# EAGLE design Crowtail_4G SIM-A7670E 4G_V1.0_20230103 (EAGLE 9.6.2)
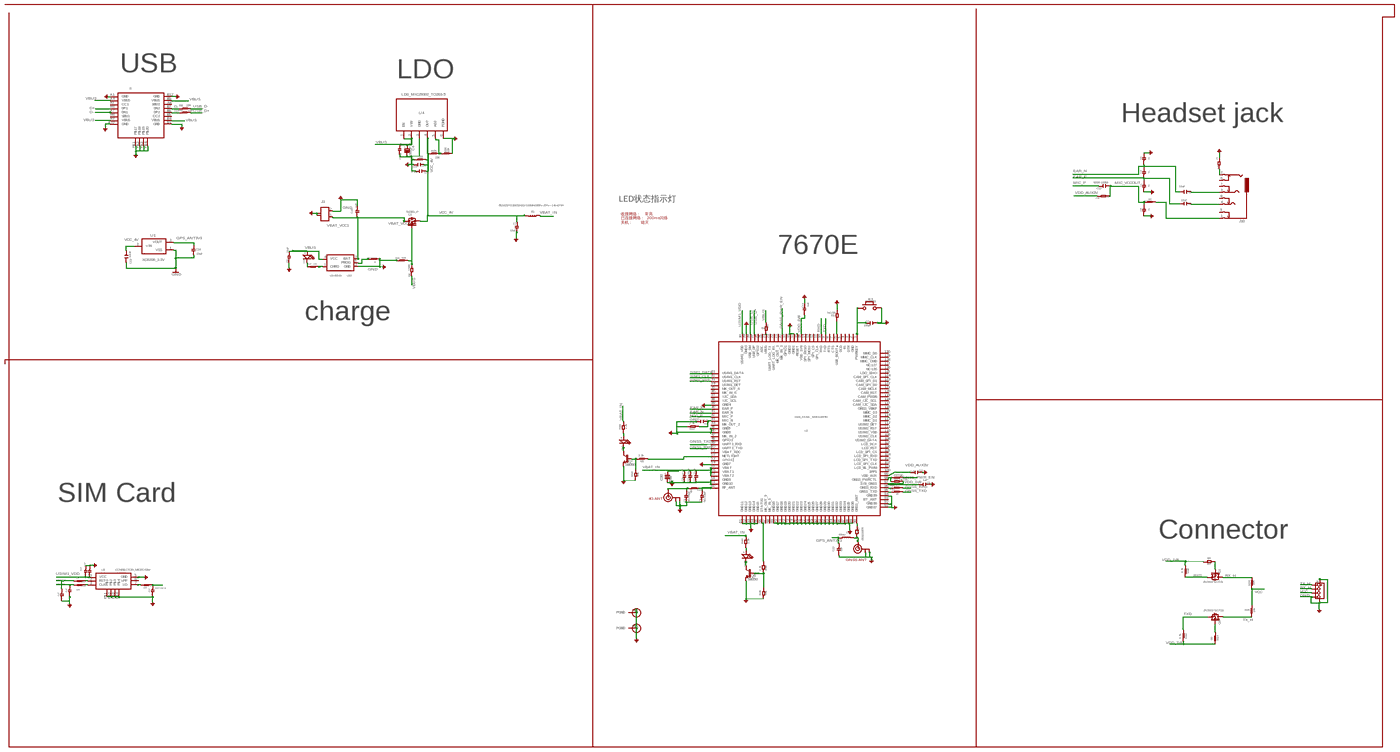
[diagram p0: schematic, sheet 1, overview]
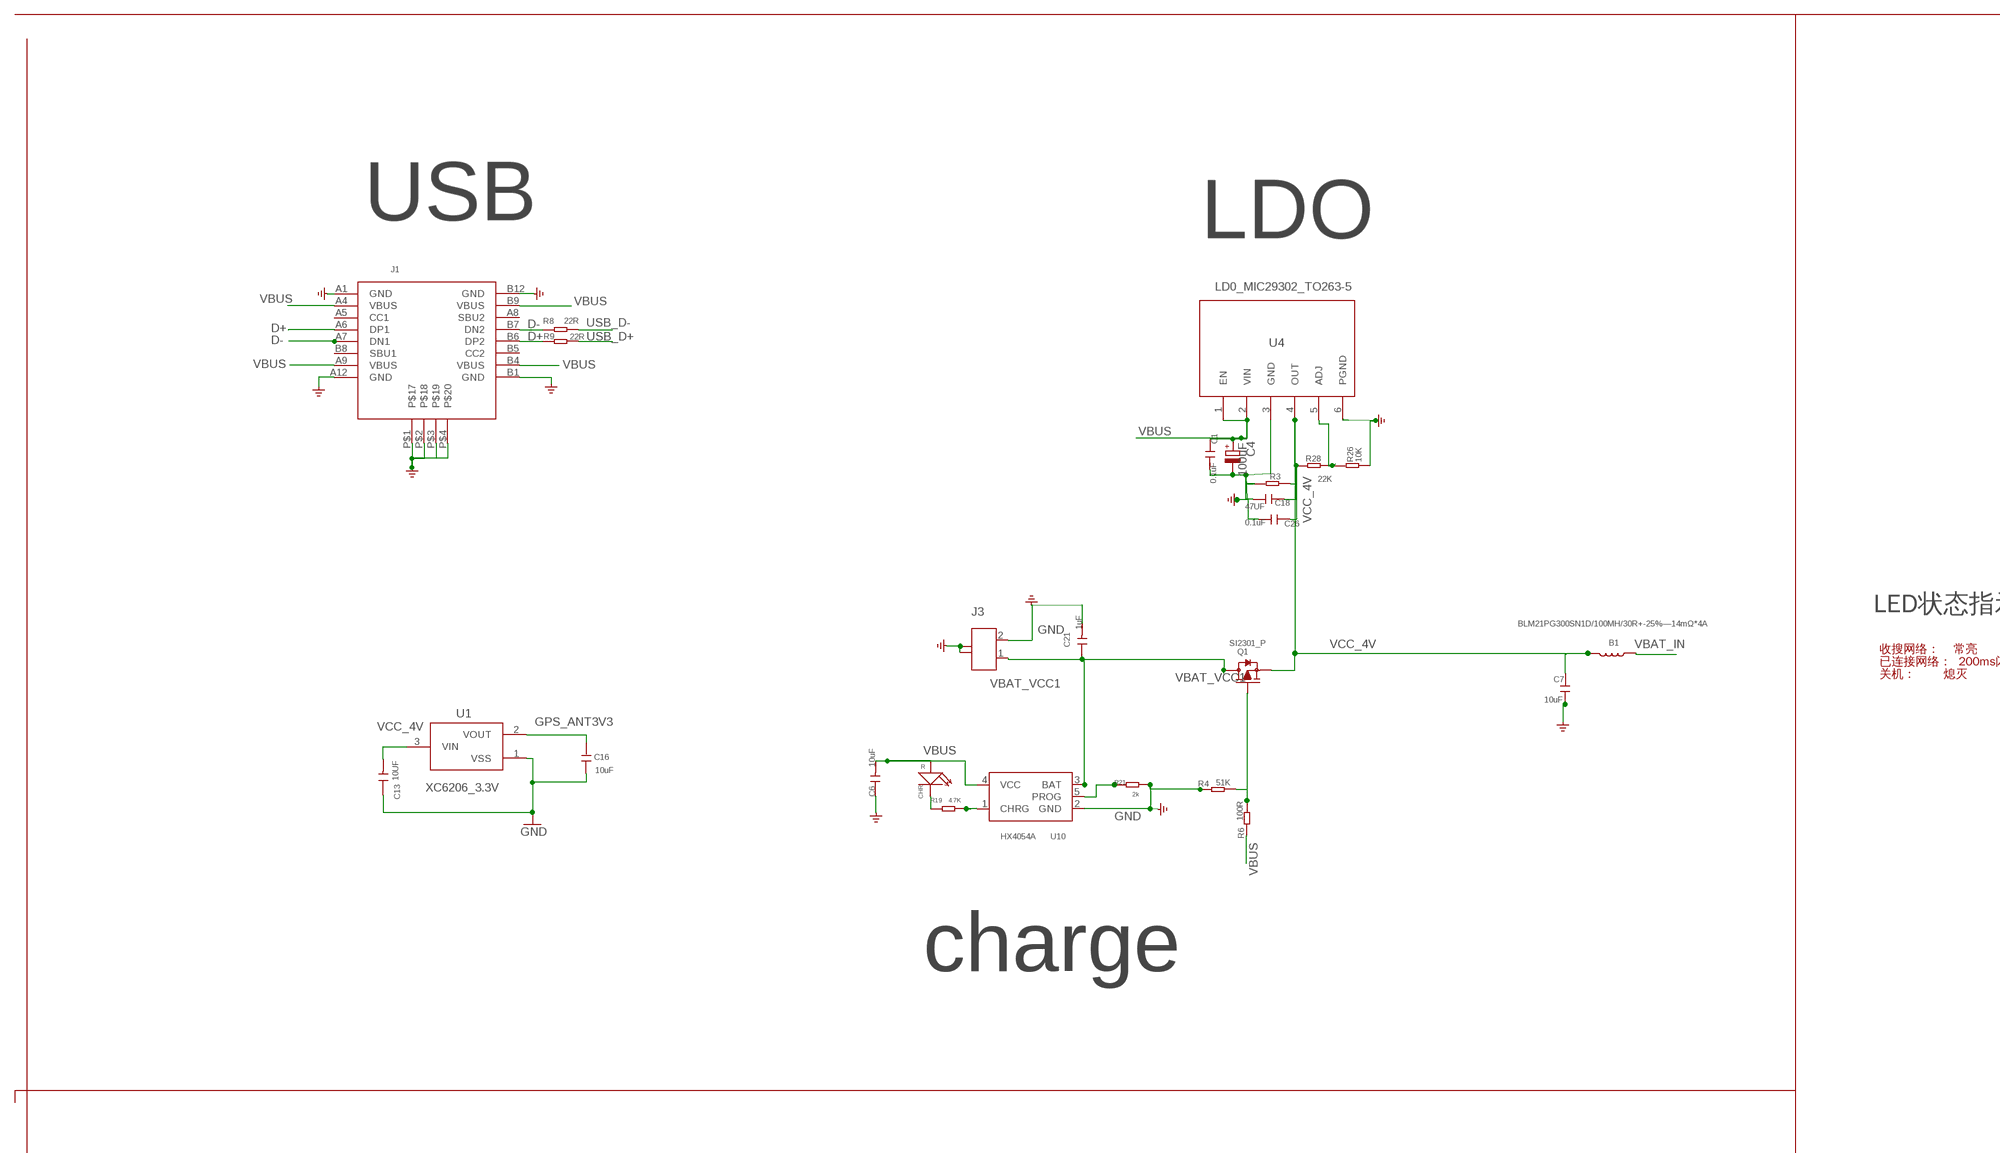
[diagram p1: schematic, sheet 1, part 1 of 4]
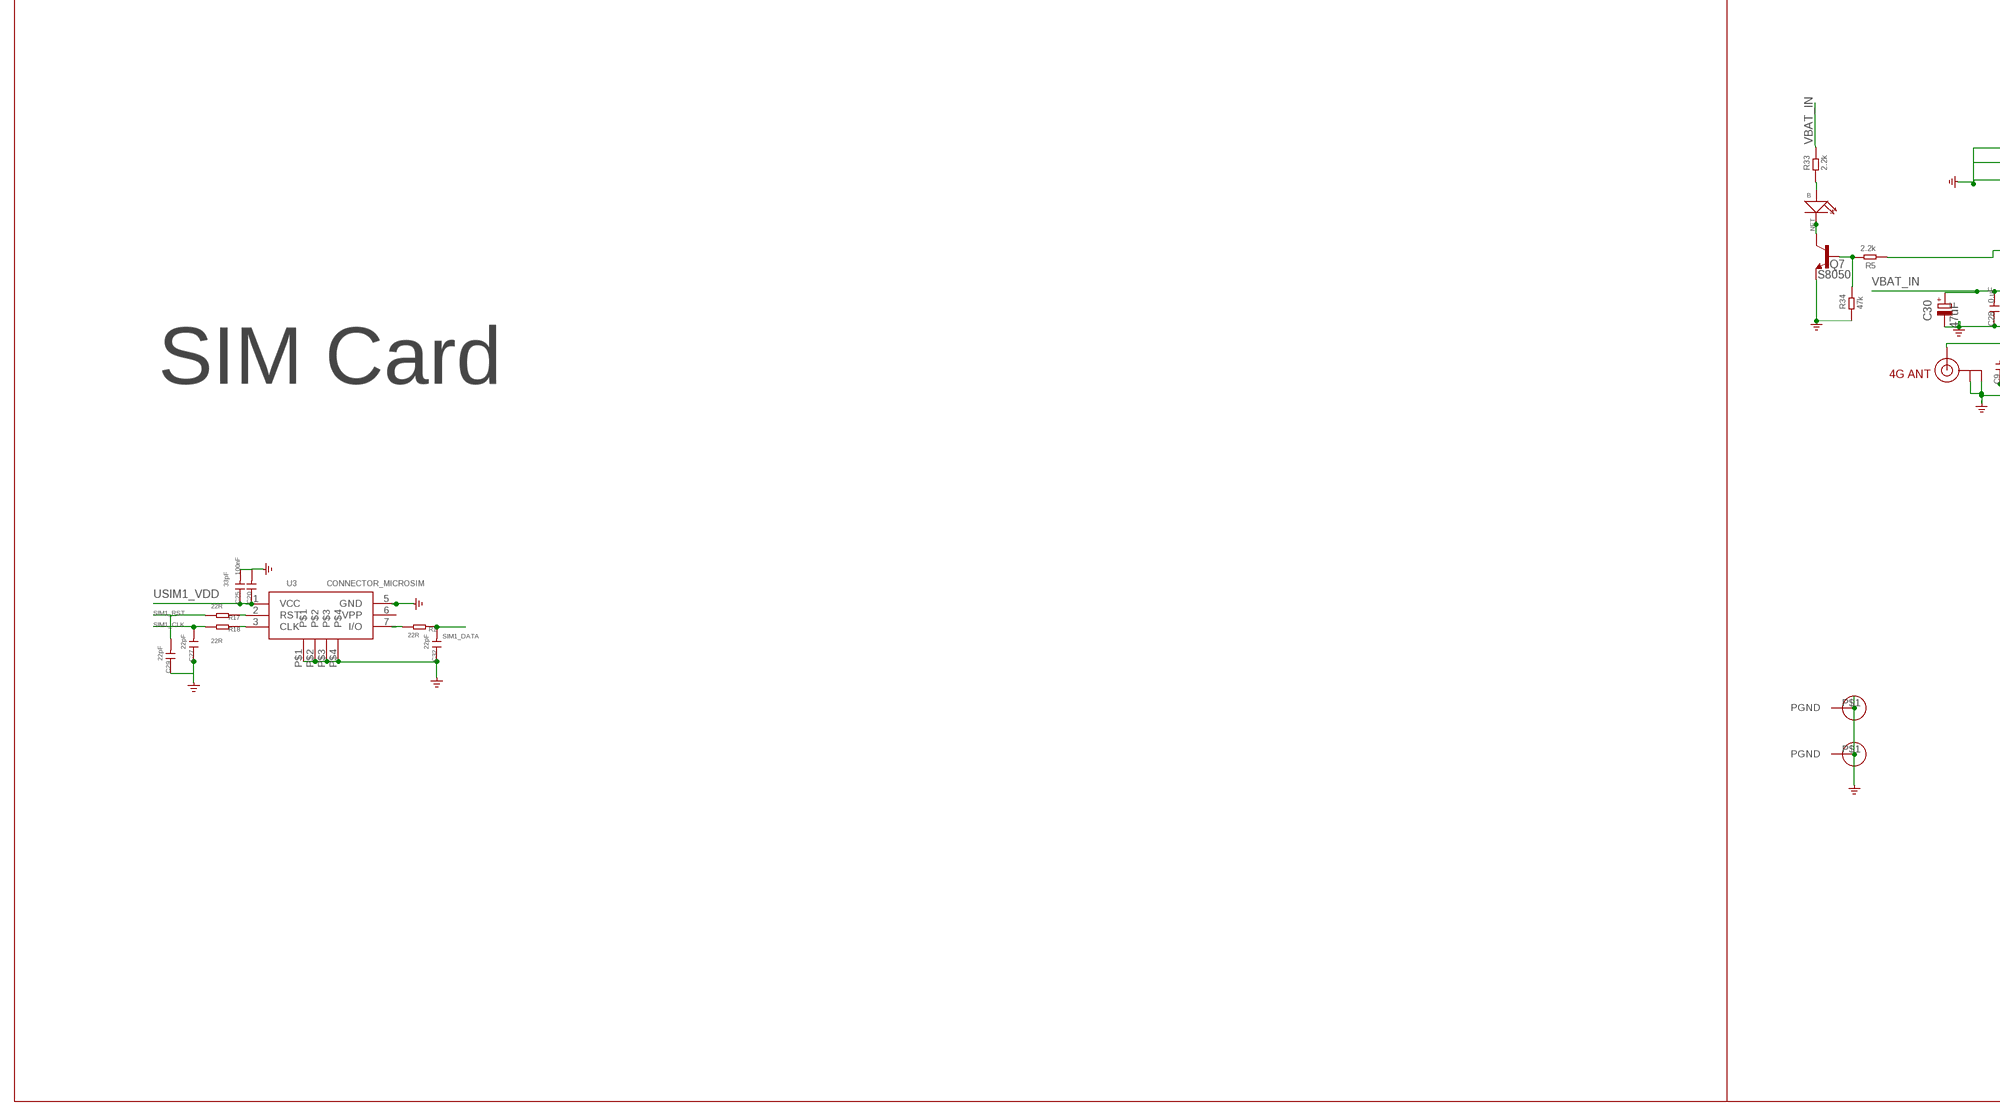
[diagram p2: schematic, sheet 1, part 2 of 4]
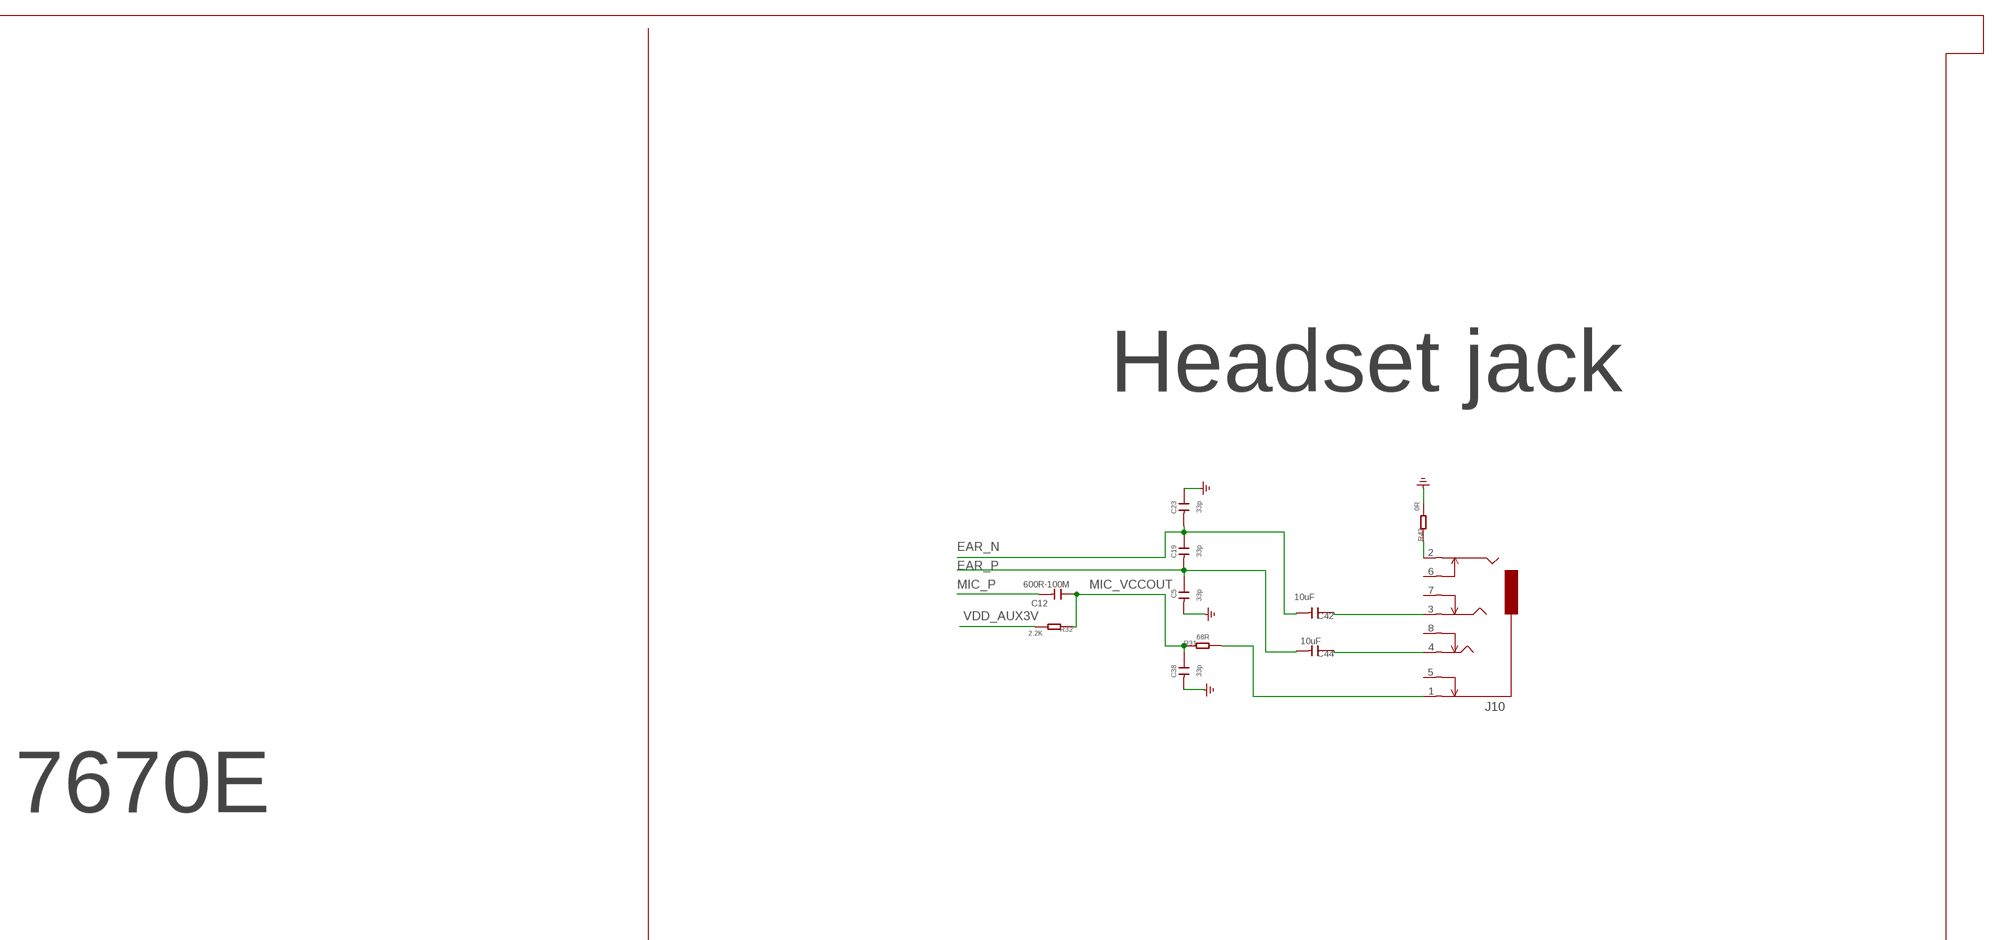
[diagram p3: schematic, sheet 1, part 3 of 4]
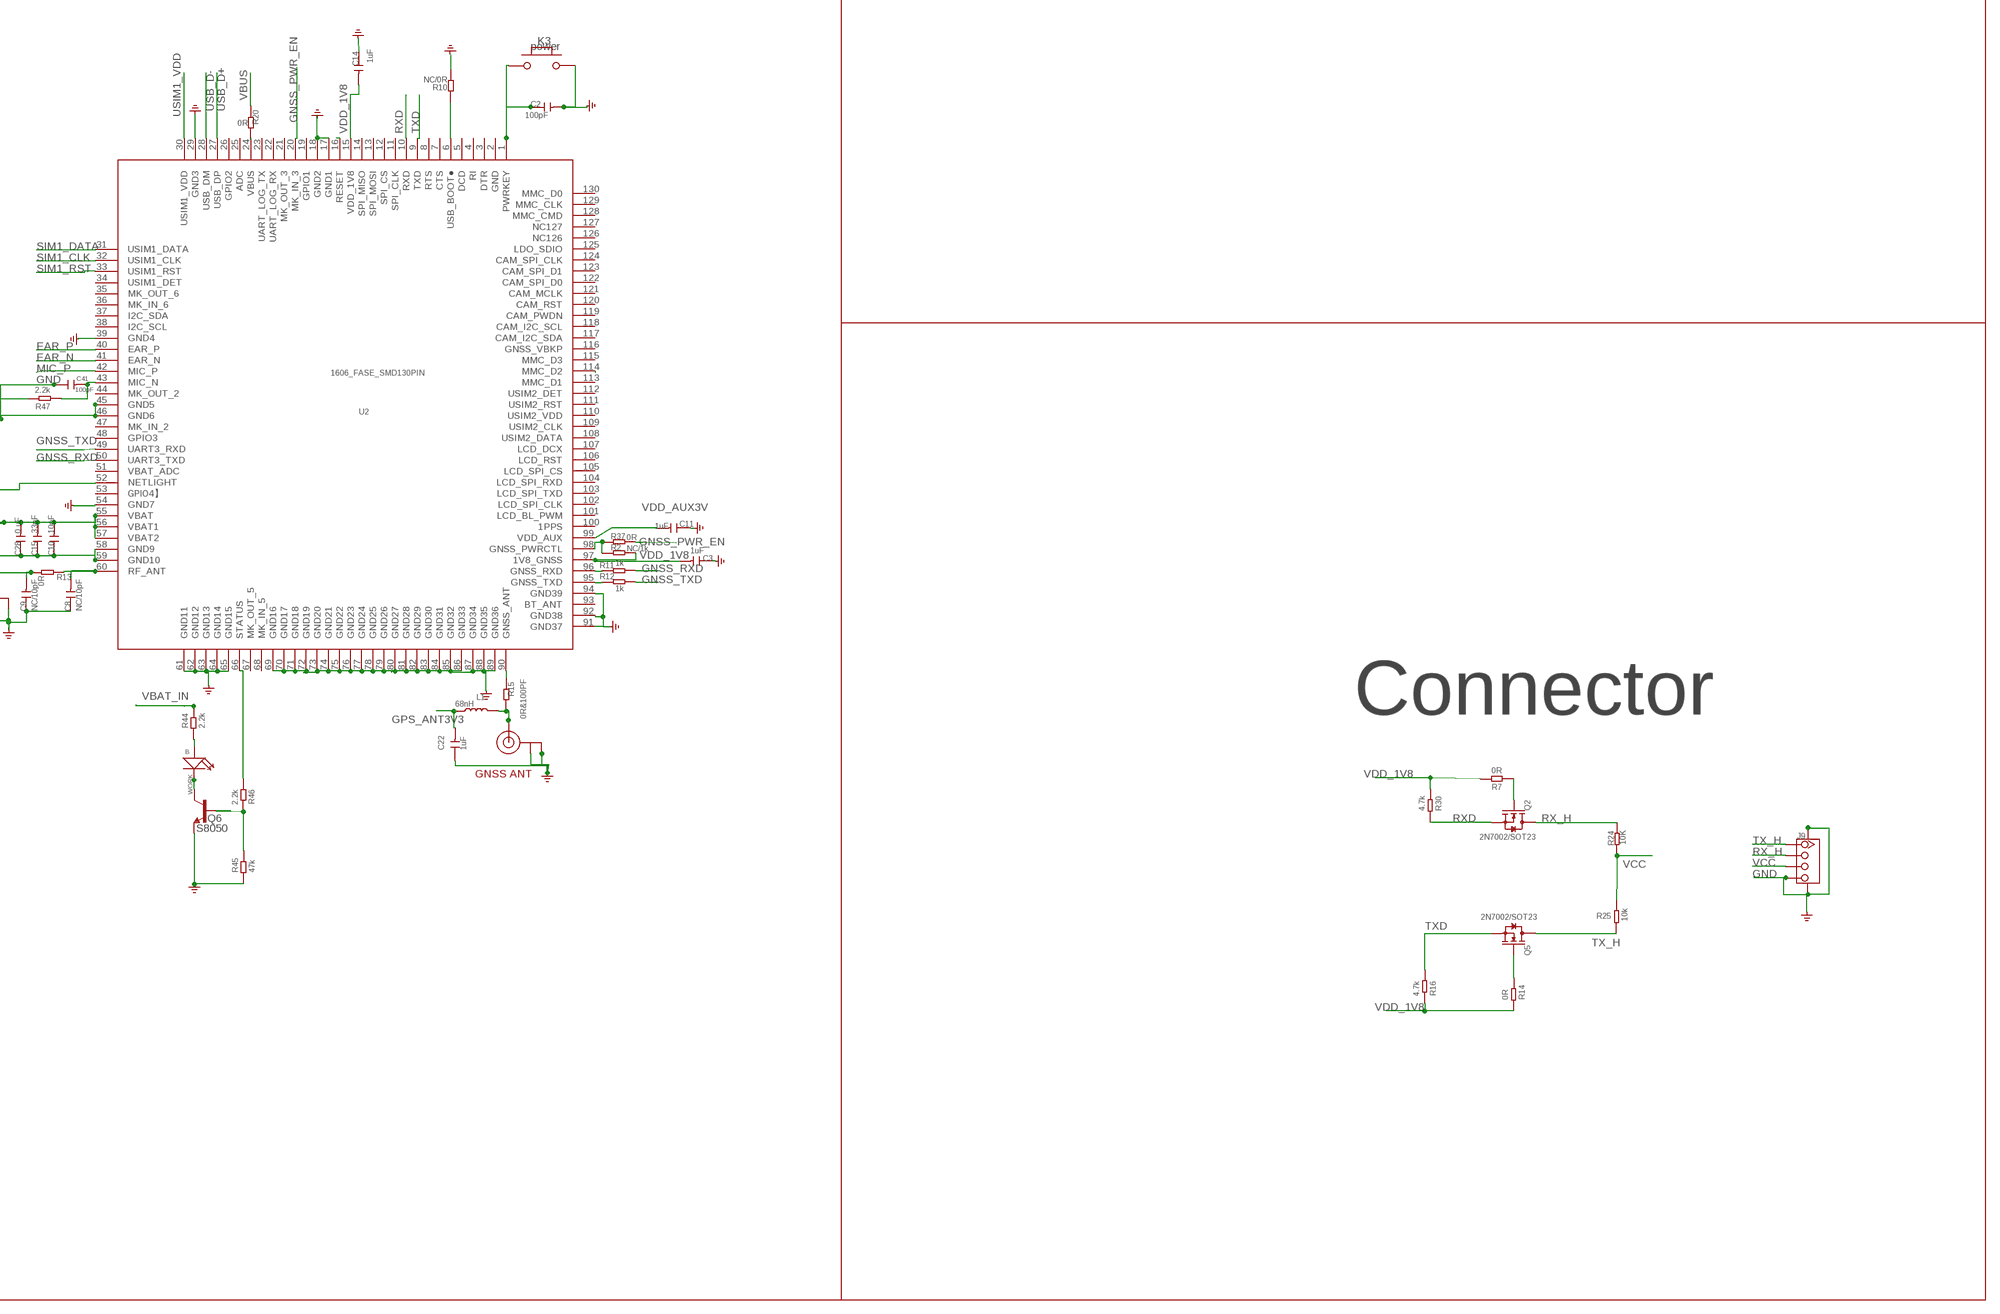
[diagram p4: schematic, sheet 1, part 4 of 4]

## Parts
B1  BLM21PG300SN1D/100MH/30R+-25%—14mΩ*4A  L0805  [0805@1]
C1  0.1uF  C0603  [0603]
C2  100pF  C-0603  [C0603]
C3  1uF  C-0603  [C0603]
C4  100uF  CPOL-EUSMCB  [SMC_B]
C5  33p  C-0603  [C0603]
C6  10uF  C-0603  [C0603]
C7  10uF  C0603  [0603]
C8  NC/10pF  C-0603  [C0603]
C9  NC/10pF  C-0603  [C0603]
C10  10pF  C-0603  [C0603]
C11  1uF  C-0603  [C0603]
C12  600R-100M  C-0603  [C0603]
C13  10UF  C-0603  [C0603]
C14  1uF  C-0603  [C0603]
C15  33pF  C-0603  [C0603]
C16  10uF  C0603  [0603]
C18  47UF  C0805  [0805]
C19  33p  C-0603  [C0603]
C20  100nF  C-0603  [C0603]
C21  1uF  C-0603  [C0603]
C22  1uF  C-0603  [C0603]
C23  33p  C-0603  [C0603]
C25  33pF  C-0603  [C0603]
C26  0.1uF  C0603  [0603]
C27  22pF  C-0603  [C0603]
C28  0.uF  C-0603  [C0603]
C29  22pF  C-0603  [C0603]
C30  47uF  CPOL-EUSMCB  [SMC_B]
C32  22pF  C-0603  [C0603]
C38  33p  C-0603  [C0603]
C41  100pF  C-0603  [C0603]
C42  10uF  C-0603  [C0603]
C44  10uF  C-0603  [C0603]
CHR  R  007-LED0603  [D0603]
J1  TYPEC-3.0-16P-SMD  [TYPEC-3.0-16P-SMD]
J3  PH2.0_2P  [PH2.0_2P]
J4  IPEX一代  U.FL  [U.FL]
J6  IPEX一代  U.FL  [U.FL]
J9  TWIG-4P-2.0-SMD-FEMALE-REINFORCE'DD'  [4P-SMD-2.0]
J10  AUDIO-8P'PJ-3536-L6S'  [8P-3.5-SMD]
K3  BUTTON  PB157  [157SW]
L1  68nH  BL_0603  [BL_0603]
NET  B  007-LED0603  [D0603]
Q1  SI2301_P  DISCRETE_MOSFET-PSOT23  [DISCRETE_SOT23]
Q2  2N7002/SOT23  MOSFET-N'SOT23'  [SOT23]
Q5  2N7002/SOT23  MOSFET-N'SOT23'  [SOT23]
Q6  S8050  SPARKFUN_TRANSISTOR_NPNSOT23  [SPARKFUN_SOT23]
Q7  S8050  SPARKFUN_TRANSISTOR_NPNSOT23  [SPARKFUN_SOT23]
R1  22R  R-0603  [R0603]
R2  NC/1k  DISCRETE_R-0603  [DISCRETE_R0603]
R3  NC/470R  DISCRETE_R-0603  [DISCRETE_R0603]
R4  51K  R0603  [R0603]
R5  2.2k  DISCRETE_R-0603  [DISCRETE_R0603]
R6  100R  R0603  [R0603]
R7  0R  R-0603  [R0603]
R8  22R  DISCRETE_R-0603  [DISCRETE_R0603]
R9  22R  DISCRETE_R-0603  [DISCRETE_R0603]
R10  NC/0R  DISCRETE_R-0603  [DISCRETE_R0603]
R11  1k  DISCRETE_R-0603  [DISCRETE_R0603]
R12  1k  DISCRETE_R-0603  [DISCRETE_R0603]
R13  0R  DISCRETE_R-0603  [DISCRETE_R0603]
R14  0R  R-0603  [R0603]
R15  0R&100PF  DISCRETE_R-0603  [DISCRETE_R0603]
R16  4.7k  R-0603  [R0603]
R17  22R  R-0603  [R0603]
R18  22R  R-0603  [R0603]
R19  4.7K  R-0603  [R0603]
R20  0R  DISCRETE_R-0603  [DISCRETE_R0603]
R21  2k  R-0603  [R0603]
R24  10K  R-0603  [R0603]
R25  10k  R-0603  [R0603]
R26  10K  DISCRETE_R-0603  [DISCRETE_R0603]
R28  22K  DISCRETE_R-0603  [DISCRETE_R0603]
R30  4.7k  R-0603  [R0603]
R31  68R  R-0603  [R0603]
R32  2.2K  R-0603  [R0603]
R33  2.2k  DISCRETE_R-0603  [DISCRETE_R0603]
R34  47k  DISCRETE_R-0603  [DISCRETE_R0603]
R37  0R  DISCRETE_R-0603  [DISCRETE_R0603]
R42  0R  R-0603  [R0603]
R44  2.2k  DISCRETE_R-0603  [DISCRETE_R0603]
R45  47k  DISCRETE_R-0603  [DISCRETE_R0603]
R46  2.2k  DISCRETE_R-0603  [DISCRETE_R0603]
R47  2.2k  DISCRETE_R-0603  [DISCRETE_R0603]
U1  XC6206_3.3V  XC6206  [SOT-23]
U2  1606_FASE_SMD130PIN  [1606_FASE_SMD130PIN]
U3  CONNECTOR_MICROSIM  [CONNECTOR_MICROSIM]
U4  LD0_MIC29302_TO263-5  [LD0_MIC29302_TO263-5]
U10  HX4054A  [HX4054A_SOT23_5]
U$37  PGND  [PGND]
U$38  PGND  [PGND]
WORK  B  007-LED0603  [D0603]

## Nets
D+: J1.A6(DP1) J1.B6(DP2) R9.1
D-: J1.A7(DN1) J1.B7(DN2) R8.1
EAR_N: C19.1 C23.2 C42.2 U2.41(EAR_N)
EAR_P: C5.1 C19.2 C44.2 U2.40(EAR_P)
GND: C1.1 C2.2 C3.1 C4.- C5.2 C6.1 C7.2 C8.1 C9.1 C10.1 C11.1 C13.1 C14.1 C15.1 C16.2 C18.1 C20.2 C21.2 C22.1 C23.1 C25.2 C26.1 C27.1 C28.1 C29.1 C30.- C32.1 C38.2 C41.1 J1.A1(GND) J1.A12(GND) J1.B1(GND) J1.B12(GND) J1.P$1 J1.P$2 J1.P$3 J1.P$4 J3.2 J3.3 J3.4 J4.P$1(GND) J4.P$2(GND) J6.P$1(GND) J6.P$2(GND) J9.4 J9.SS1 J9.SS2 K3.2 Q6.2(E) Q7.2(E) R3.2 R4.2 R10.2 R21.2 R26.2 R34.1 R42.2 R45.1 R47.2 U1.1(VSS) U2.17(GND1) U2.18(GND2) U2.29(GND3) U2.39(GND4) U2.45(GND5) U2.46(GND6) U2.54(GND7) U2.58(GND9) U2.59(GND10) U2.61(GND11) U2.62(GND12) U2.63(GND13) U2.64(GND14) U2.65(GND15) U2.69(GND16) U2.70(GND17) U2.71(GND18) U2.72(GND19) U2.73(GND20) U2.74(GND21) U2.75(GND22) U2.76(GND23) U2.77(GND24) U2.78(GND25) U2.79(GND26) U2.80(GND27) U2.81(GND28) U2.82(GND29) U2.83(GND30) U2.84(GND31) U2.85(GND32) U2.86(GND33) U2.87(GND34) U2.88(GND35) U2.89(GND36) U2.91(GND37) U2.92(GND38) U2.94(GND39) U3.5(GND) U3.P$1 U3.P$2 U3.P$3 U3.P$4 U4.3(GND) U4.6(PGND) U10.2(GND) U$37.P$1(PGND) U$38.P$1(PGND)
GNSS_PWR_EN: R37.2 U2.20(MK_IN_3)
GNSS_RXD: R11.2 U2.50(UART3_TXD)
GNSS_TXD: R12.2 U2.49(UART3_RXD)
GPS_ANT3V3: C16.1 C22.2 L1.1 U1.2(VOUT)
MIC_P: C12.2 U2.42(MIC_P)
MIC_VCCOUT: C12.1 C38.1 R31.1 R32.1
N$1: R18.1 U3.3(CLK)
N$2: R17.1 U3.2(RST)
N$3: Q1.1(G) R4.1 R6.1
N$4: Q2.1(G) R7.2
N$5: R5.1 U2.52(NETLIGHT)
N$6: U2.16(RESET)
N$7: CHR.- R19.1
N$8: R10.1 U2.6(USB_BOOT●)
N$9 [N9]: J4.P$3(SIGNAL) L1.2 R15.2
N$10: R12.1 U2.95(GNSS_TXD)
N$11: Q5.1(G) R14.2
N$12: R11.1 U2.96(GNSS_RXD)
N$13 [N13]: C8.2 R13.1 U2.60(RF_ANT)
N$15 [N15]: C9.2 J6.P$3(SIGNAL) R13.2
N$16 [N16]: R15.1 U2.90(GNSS_ANT)
N$17: Q7.1(B) R5.2 R34.2
N$18: C41.2 R47.1 U2.43(MIC_N)
N$20: R19.2 U10.1(CHRG)
N$21: J10.1 R31.2
N$22: R26.1 R28.1 U4.5(ADJ)
N$23: J10.2 R42.1
N$24: R1.2 U3.7(I/O)
N$25: R20.2 U2.24(VBUS)
N$26: C42.1 J10.3
N$27: C44.1 J10.4
N$29: R2.1 R37.1 U2.98(GNSS_PWRCTL)
N$31: R21.1 U10.5(PROG)
N$32: C2.1 K3.1 U2.1(PWRKEY)
N$35: NET.- Q7.3(C)
N$36: NET.+ R33.1
N$37: Q6.1(B) R45.2 R46.2
N$39: Q6.3(C) WORK.-
N$40: R44.1 WORK.+
N$41: R46.1 U2.66(STATUS)
RX_H: J9.2 Q2.3(D) R24.1
RXD: Q2.2(S) R30.1 U2.10(RXD)
SIM1_CLK: C27.2 R18.2 U2.32(USIM1_CLK)
SIM1_DATA: C32.2 R1.1 U2.31(USIM1_DATA)
SIM1_RST: C29.2 R17.2 U2.33(USIM1_RST)
TF_DAT2: U2.114(MMC_D2)
TX_H: J9.1 Q5.3(D) R25.1
TXD: Q5.2(S) R16.1 U2.9(TXD)
USB_D+: R9.2 U2.27(USB_DP)
USB_D-: R8.2 U2.28(USB_DM)
USIM1_VDD: C20.1 C25.1 U2.30(USIM1_VDD) U3.1(VCC)
VBAT_IN: B1.1 C10.2 C15.2 C28.2 C30.+ R33.2 R44.2 U2.55(VBAT) U2.56(VBAT1) U2.57(VBAT2)
VBAT_VCC1: C21.1 J3.1 Q1.3(D) U10.3(BAT)
VBUS: C1.2 C4.+ C6.2 CHR.+ J1.A4(VBUS) J1.A9(VBUS) J1.B4(VBUS) J1.B9(VBUS) R6.2 R20.1 U4.1(EN) U4.2(VIN) U10.4(VCC)
VCC: J9.3 R24.2 R25.2
VCC_4V: B1.2 C7.1 C13.2 C18.2 C26.2 Q1.2(S) R3.1 R28.2 U1.3(VIN) U4.4(OUT)
VDD_1V8: C3.2 C14.2 R2.2 R7.1 R14.1 R16.2 R30.2 U2.15(VDD_1V8) U2.97(1V8_GNSS)
VDD_AUX3V: C11.2 R32.2 U2.99(VDD_AUX)
Unconnected: J1.A5(CC1) J1.A8(SBU2) J1.B5(CC2) J1.B8(SBU1) J10.5 J10.6 J10.7 J10.8 U2.2(GND) U2.3(DTR) U2.4(RI) U2.5(DCD) U2.7(CTS) U2.8(RTS) U2.11(SPI_CLK) U2.12(SPI_CS) U2.13(SPI_MOSI) U2.14(SPI_MISO) U2.19(GPIO1) U2.21(MK_OUT_3) U2.22(UART_LOG_RX) U2.23(UART_LOG_TX) U2.25(ADC) U2.26(GPIO2) U2.34(USIM1_DET) U2.35(MK_OUT_6) U2.36(MK_IN_6) U2.37(I2C_SDA) U2.38(I2C_SCL) U2.44(MK_OUT_2) U2.47(MK_IN_2) U2.48(GPIO3) U2.51(VBAT_ADC) U2.53(GPIO4】) U2.67(MK_OUT_5) U2.68(MK_IN_5) U2.93(BT_ANT) U2.100(1PPS) U2.101(LCD_BL_PWM) U2.102(LCD_SPI_CLK) U2.103(LCD_SPI_TXD) U2.104(LCD_SPI_RXD) U2.105(LCD_SPI_CS) U2.106(LCD_RST) U2.107(LCD_DCX) U2.108(USIM2_DATA) U2.109(USIM2_CLK) U2.110(USIM2_VDD) U2.111(USIM2_RST) U2.112(USIM2_DET) U2.113(MMC_D1) U2.115(MMC_D3) U2.116(GNSS_VBKP) U2.117(CAM_I2C_SDA) U2.118(CAM_I2C_SCL) U2.119(CAM_PWDN) U2.120(CAM_RST) U2.121(CAM_MCLK) U2.122(CAM_SPI_D0) U2.123(CAM_SPI_D1) U2.124(CAM_SPI_CLK) U2.125(LDO_SDIO) U2.126(NC126) U2.127(NC127) U2.128(MMC_CMD) U2.129(MMC_CLK) U2.130(MMC_D0) U3.6(VPP)

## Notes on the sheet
- USB | LDO
- Headset jack
- LED状态指示灯
- 收搜网络：    常亮 
  已连接网络：  200ms闪烁
  关机：        熄灭
- 7670E
- power
- charge
- 4G ANT
- SIM Card
- Connector
- GNSS ANT

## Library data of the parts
B1 = Discrete:L*
C1 C7 C16 C26 = cooper:C0603
C2 C3 C5 C6 C8-C15 C19-C23 C25 C27-C29 C32 C38 C41 C42 C44 = Discrete:C*: Ceramic Capacitors
C4 C30 = rcl:CPOL-EU: POLARIZED CAPACITOR, European symbol
C18 = cooper:C0805
CHR NET WORK = Discrete:007-LED*
J1 = A_xbj:TYPEC-3.0-16P-SMD
J3 = A_xbj:PH2.0_2P
J4 J6 = SparkFun2:U.FL
J9 = Connector:TWIG-4P-2.0-SMD-FEMALE-REINFORCE
J10 = template:AUDIO-8P
K3 = MySMD:PB157
L1 = untitled:BL_0603
Q1 = untitled:DISCRETE_MOSFET-P: IRLL014: http://www.vishay.com/docs/91319/sihll014.pdf
Q2 Q5 = Discrete:MOSFET-N: IRLL014: http://www.vishay.com/docs/91319/sihll014.pdf
Q6 Q7 = Adafruit_HUZZAH32_ESP32_Feather:SPARKFUN_TRANSISTOR_NPN: Transistor NPN BJT configuration in SOT23 package. MMBT2222 is the common NPN we use. Double check BCE configuration again layout.
R1 R7 R14 R16-R19 R21 R24 R25 R30-R32 R42 = Discrete:R*
R2 R5 R8 R9 R11 R12 R33 R34 R37 R44-R47 = Crowtail-_LED-V2.0-20190615-01:DISCRETE_R*
R3 R10 R13 R15 R20 R26 R28 = A9G:DISCRETE_R*
R4 R6 = cooper:R0603
U1 = self:XC6206
U2 = A7670E_FASE_SMD124PIN:1606_FASE_SMD130PIN
U3 = MINISIM_MUPC713-23_6PIN:CONNECTOR_MICROSIM
U4 = LD0_MIC29302_TO263-5:LD0_MIC29302_TO263-5
U10 = ESP32-S3-WROOM-2-N32R8V1:HX4054A
U$37 U$38 = QC:PGND

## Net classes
0 default: width 0.152 mm, drill 0.3 mm, clearance 0.152 mm
1 N9: drill 0.533 mm, clearance 0.533 mm to class 0, clearance 0.533 mm
2 N13: drill 0.533 mm, clearance 0.533 mm to class 0, clearance 0.533 mm
3 N15: drill 0.533 mm, clearance 0.533 mm to class 0, clearance 0.533 mm
4 N16: clearance 0.254 mm to class 0, clearance 0.254 mm

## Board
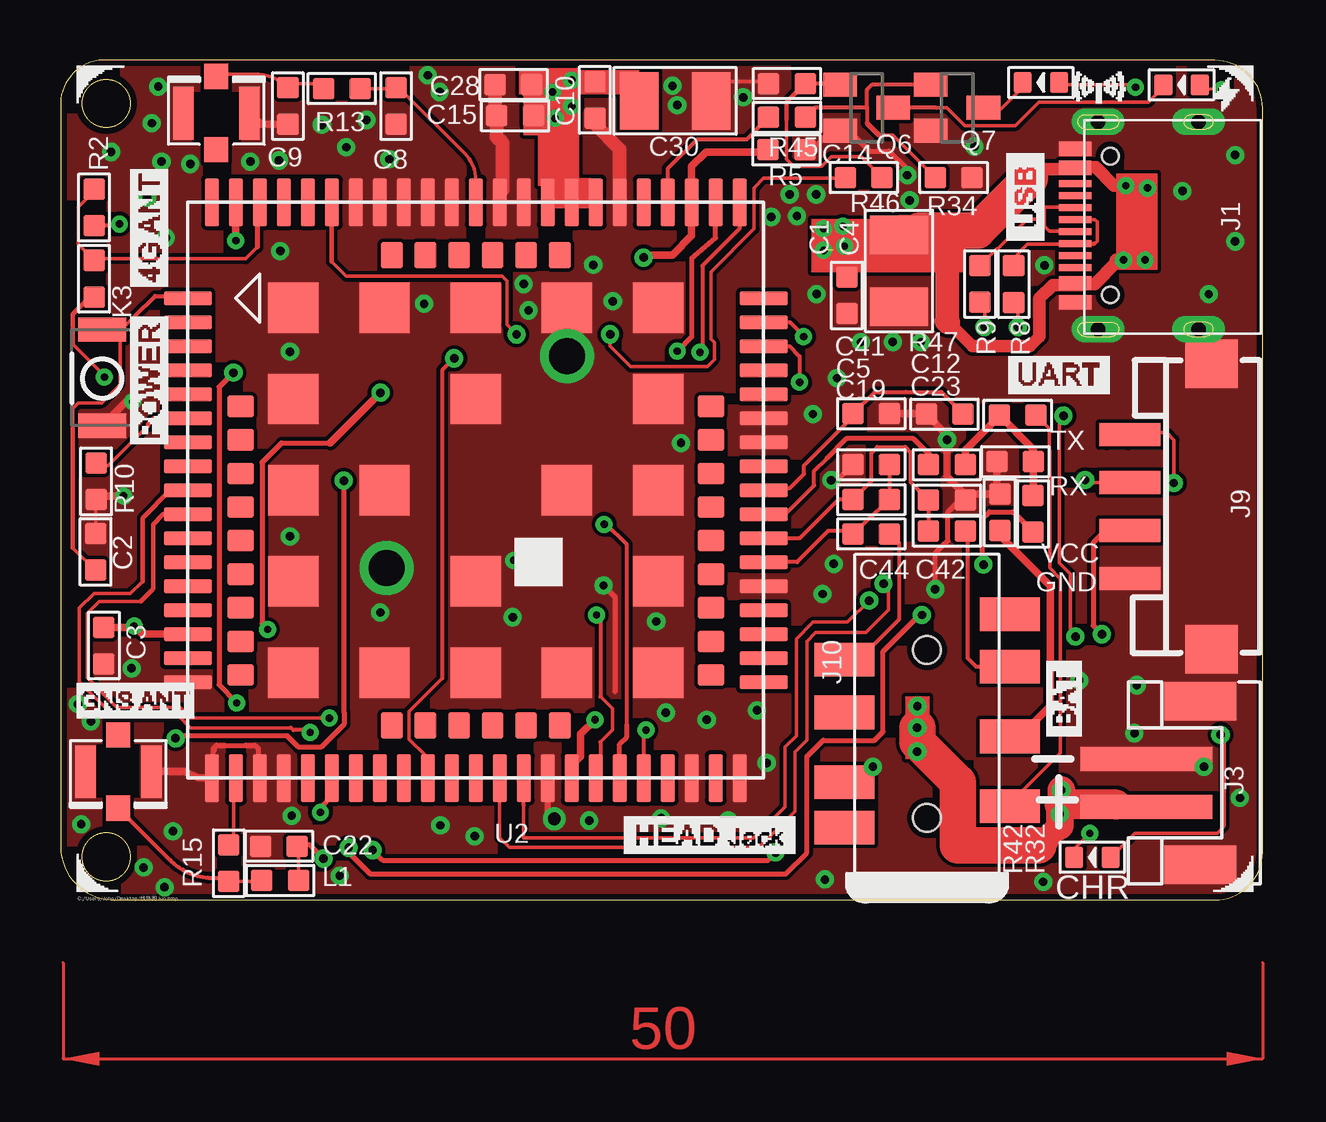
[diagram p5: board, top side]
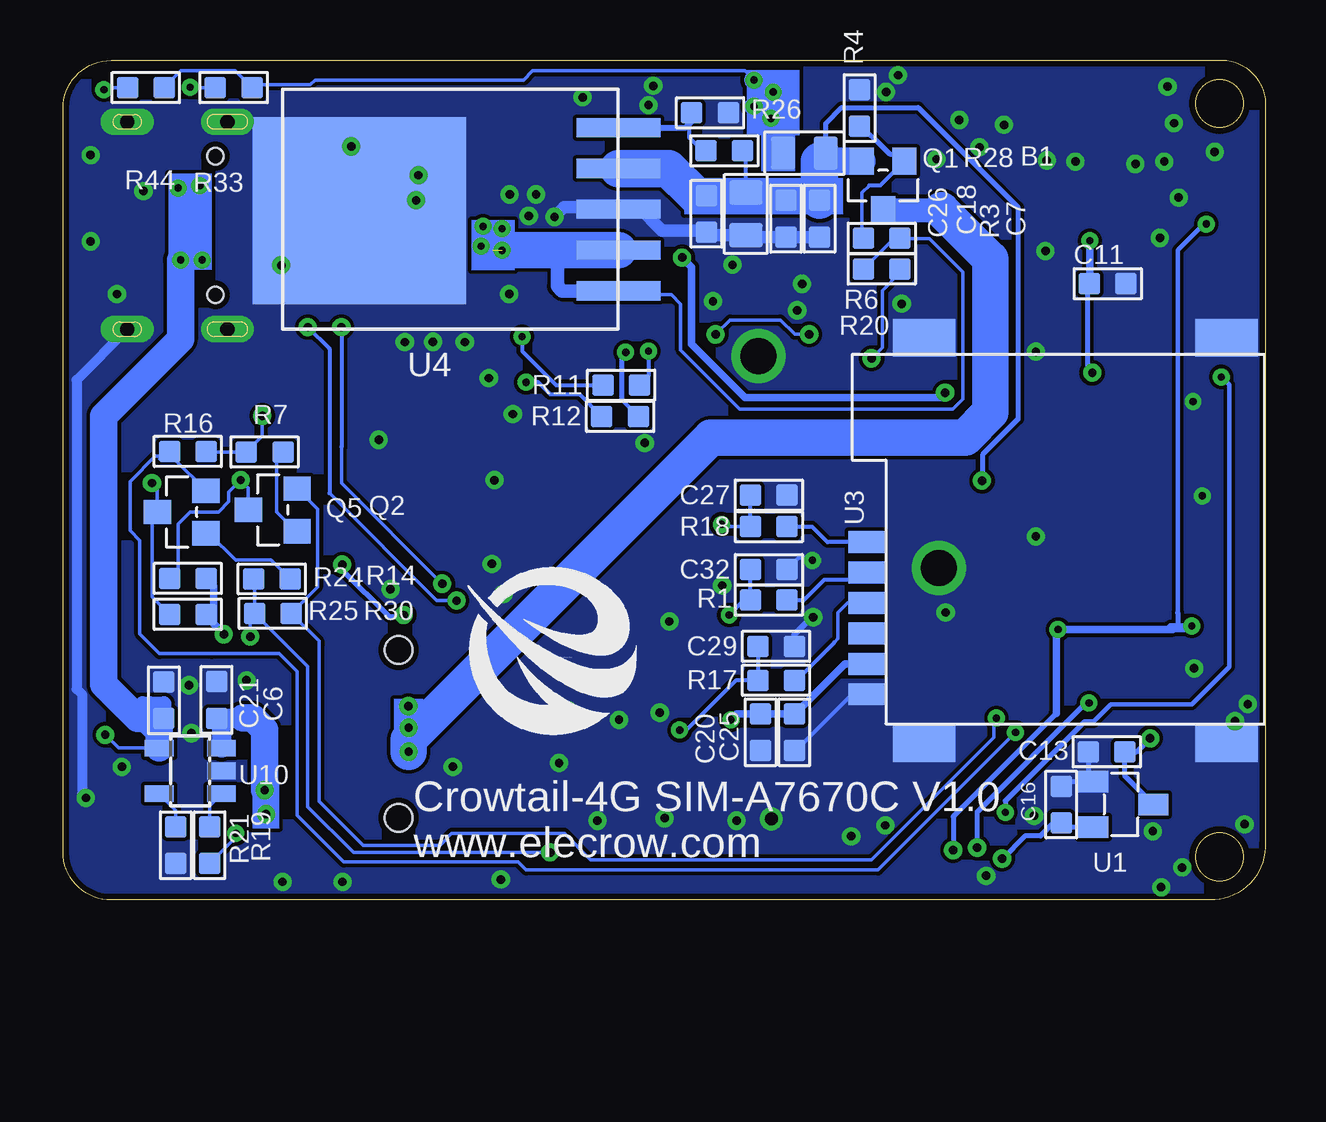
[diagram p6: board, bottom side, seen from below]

Size 50.1 x 35.02 mm. Coordinates in mm from the lower left corner, seen from the top.
Outline: 0,33.4 0,2.4 arc90 2.1,0 48.1,0 arc90 50.1,2 50.1,33 arc90 48.1,35 2.1,35 arc90 0,33.4
Outline: circle at 1.9,33.2 radius 1
Outline: circle at 1.9,1.8 radius 1
Copper layers (1*16): Top 0.035mm / dielectric 1.5mm / Bottom 0.035mm
Design rules "default *": minimum track width 6mil, minimum drill 0.3mm, track to track 6mil, track to pad 6mil, pad to pad 6mil, via to via 6mil, smd to smd 6mil, copper to edge 10mil, drill to drill 6mil, minimum pad ring 10mil, minimum via ring 8mil, stop-mask expansion 4mil, vias tented up to drill 40mil, thermal gap 10mil
tRestrict: area 5.5,31.5 to 7.5,33.7; area 1.5,4.3 to 3.3,6.5

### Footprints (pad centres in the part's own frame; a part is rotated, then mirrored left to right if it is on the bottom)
0805@1 = smd 1.016 x 1.397: 1 -0.889,0; 2 0.889,0
0603 = smd 0.889 x 0.889: 1 -0.762,0; 2 0.762,0
C0603 = smd 0.889 x 0.889: 1 -0.762,0; 2 0.762,0
SMC_B = smd 1.6 x 2.4: + -1.5,0; - 1.5,0
0805 = smd 1.016 x 1.397: 1 -0.889,0; 2 0.889,0
D0603 = smd 0.762 x 0.889: + -0.762,0; - 0.762,0
TYPEC-3.0-16P-SMD = smd 0.3 x 1.35: A1 -3.35,0.25; A4 -2.55,0.25; A5 -1.25,0.25; A6 -0.25,0.25; A7 0.25,0.25; A8 -1.75,0.25; A9 2.55,0.25; A12 3.35,0.25; B1 3.05,0.25; B4 2.25,0.25; B5 1.75,0.25; B6 0.75,0.25; B7 -0.75,0.25; B8 1.25,0.25; B9 -2.25,0.25; B12 -3.05,0.25 | drill 0.6 pad 1.016 long: P$1 -4.325,-0.72; P$2 4.325,-0.72; P$3 -4.325,-4.9; P$4 4.325,-4.9 | hole 0.68: -2.89,-1.22; 2.89,-1.22
PH2.0_2P = smd 1 x 5.5: 1 -1,2.75; 2 1,2.75 | smd 1.6 x 3: 3 -3.4,0.5; 4 3.4,0.5
U.FL = smd 2.2 x 0.85: P$1 0,1.375; P$2 0,-1.375 | smd 1.05 x 1: P$3 1.525,0; P$4 -1.525,0
4P-SMD-2.0 = smd 0.965 x 2.54: 1 -3,0; 2 -1,0; 3 1,0; 4 3,0 | smd 2.032 x 2.184: SS1 -5.946,3.4; SS2 5.946,3.4
8P-3.5-SMD = smd 1.4 x 2.5: 1 2.8,-3.45; 2 5.7,-3.45; 3 8.6,-3.45; 4 8.9,3.45; 5 1.9,3.45; 6 3.8,3.45; 7 6.7,3.45; 8 10.8,-3.45 | hole 1.149: 2.3,0; 9.3,0
157SW = smd 1.016 x 1.981: 1 0,0; 2 4,0
BL_0603 = smd 0.889 x 0.889: 1 -0.762,0; 2 0.762,0
DISCRETE_SOT23 = smd 1.016 x 1.143: 1 -0.889,-1.016; 2 0.889,-1.016; 3 0,1.016
SOT23 = smd 1.016 x 1.143: 1 -0.889,-1.016; 2 0.889,-1.016; 3 0,1.016
SPARKFUN_SOT23 = smd 1 x 1.4: 1 -0.95,-1.1; 2 0.95,-1.1; 3 0,1.1
R0603 = smd 0.889 x 0.889: 1 -0.762,0; 2 0.762,0
DISCRETE_R0603 = smd 0.889 x 0.889: 1 -0.762,0; 2 0.762,0
SOT-23 = smd 0.9 x 1.25: 1 -0.95,-1.25; 2 0.95,-1.25; 3 0,1.25
1606_FASE_SMD130PIN = smd 2 x 0.6: 1 -12,8; 2 -12,7; 3 -12,6; 4 -12,5; 5 -12,4; 6 -12,3; 7 -12,2; 8 -12,1; 9 -12,0; 10 -12,-1; 11 -12,-2; 12 -12,-3; 13 -12,-4; 14 -12,-5; 15 -12,-6; 16 -12,-7; 17 -12,-8; 35 12,-8; 36 12,-7; 37 12,-6; 38 12,-5; 39 12,-4; 40 12,-3; 41 12,-2; 42 12,-1; 43 12,0; 44 12,1; 45 12,2; 46 12,3; 47 12,4; 48 12,5; 49 12,6; 50 12,7; 51 12,8 | smd 0.6 x 2: 18 -8,-12; 19 -7,-12; 20 -6,-12; 21 -5,-12; 22 -4,-12; 23 -3,-12; 24 -2,-12; 25 -1,-12; 26 0,-12; 27 1,-12; 28 2,-12; 29 3,-12; 30 4,-12; 31 5,-12; 32 6,-12; 33 7,-12; 34 8,-12; 52 8,12; 53 7,12; 54 6,12; 55 5,12; 56 4,12; 57 3,12; 58 2,12; 59 1,12; 60 0,12; 61 -1,12; 62 -2,12; 63 -3,12; 64 -4,12; 65 -5,12; 66 -6,12; 67 -7,12; 68 -8,12; 89 -11,-12; 90 -10,-12; 91 -9,-12; 92 9,-12; 93 10,-12; 94 11,-12; 95 11,12; 96 10,12; 97 9,12; 98 -9,12; 99 -10,12; 100 -11,12 | smd 2.1 x 2.1: 69 -7.6,7.6; 70 -7.6,3.8; 71 -7.6,0; 72 -7.6,-3.8; 73 -7.6,-7.6; 74 -3.8,-7.6; 75 0,-7.6; 76 3.8,-7.6; 77 7.6,-7.6; 78 7.6,-3.8; 79 7.6,0; 80 7.6,3.8; 81 7.6,7.6; 82 3.8,7.6; 83 0,7.6; 84 -3.8,7.6; 85 -3.8,0; 86 0,-3.8; 87 3.8,0; 88 0,3.8 | smd 1.1 x 0.9: 101 -9.8,3.5; 102 -9.8,2.1; 103 -9.8,0.7; 104 -9.8,-0.7; 105 -9.8,-2.1; 106 -9.8,-3.5; 113 9.8,-3.5; 114 9.8,-2.1; 115 9.8,-0.7; 116 9.8,0.7; 117 9.8,2.1; 118 9.8,3.5; 125 -9.8,-4.9; 126 -9.8,-6.3; 127 -9.8,-7.7; 128 9.8,-7.7; 129 9.8,-6.3; 130 9.8,-4.9 | smd 0.9 x 1.1: 107 -3.5,-9.8; 108 -2.1,-9.8; 109 -0.7,-9.8; 110 0.7,-9.8; 111 2.1,-9.8; 112 3.5,-9.8; 119 3.5,9.8; 120 2.1,9.8; 121 0.7,9.8; 122 -0.7,9.8; 123 -2.1,9.8; 124 -3.5,9.8
CONNECTOR_MICROSIM = smd 1.5 x 0.9: 1 -0.8,2.5; 2 -0.8,5.04; 3 -0.8,7.58; 5 -0.8,1.23; 6 -0.8,3.77; 7 -0.8,6.31 | smd 2.61 x 1.56: P$1 1.6,-0.8; P$2 14.2,-0.8; P$3 14.2,16.1; P$4 1.6,16.1
LD0_MIC29302_TO263-5 = smd 3.5 x 0.8: 1 0,-3.4; 2 0,-1.7; 3 0,0; 4 0,1.7; 5 0,3.4 | smd 8.9 x 7.8: 6 -10.8,-0.06
HX4054A_SOT23_5 = smd 1.2 x 0.69: 1 1.3,-0.95; 2 1.3,0; 3 1.3,0.95; 4 -1.3,0.95; 5 -1.3,-0.95
PGND = drill 1.5: P$1 0,0

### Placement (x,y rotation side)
B1  19.2,31.13 0 bottom
C1  32.77,25.2 90 top
C2  1.46,14.51 90 top
C3  1.8,10.6 90 top
C4  34.94,26.22 270 top
C5  33.79,18.15 180 top
C6  45.9,8.32 270 bottom
C7  18.57,28.4 270 bottom
C8  13.98,33.09 90 top
C9  9.47,33.09 90 top
C10  22.27,33.35 90 top
C11  6.56,25.69 180 bottom
C12  36.94,18.15 180 top
C13  6.6,6.18 0 bottom
C14  30.25,31.27 180 top
C15  18.94,32.69 0 top
C16  8.5,3.98 90 bottom
C18  21.64,28.6 90 bottom
C19  33.79,16.69 0 top
C20  21.03,6.99 270 bottom
C21  43.7,8.34 90 bottom
C22  9.1,2.24 0 top
C23  36.94,16.67 180 top
C25  19.63,6.99 270 bottom
C26  23.29,28.6 90 bottom
C27  20.69,16.87 180 bottom
C28  18.87,33.99 0 top
C29  20.39,10.57 180 bottom
C30  25.61,33.31 0 top
C32  20.69,13.77 180 bottom
C38  39.79,18.27 180 top
C41  33.79,20.27 180 top
C42  36.94,15.37 180 top
C44  33.79,15.26 180 top
CHR  43,1.78 180 top
J1  42.53,28.11 90 top
J3  48,4.88 90 top
J4  2.4,5.35 270 top
J6  6.49,32.8 90 top
J9  44.58,16.4 270 top
J10  36.12,1.12 90 top
K3  1.73,23.77 270 top
L1  9.15,0.81 180 top
NET  40.86,34.08 180 top
Q1  15.93,29.78 180 bottom
Q2  41.36,16.26 90 bottom
Q5  45.16,16.17 90 bottom
Q6  33.6,33.02 270 top
Q7  37.36,33.02 270 top
R1  20.69,12.5 0 bottom
R2  1.4,28.87 270 top
R3  19.97,28.4 270 bottom
R4  16.9,33.01 90 bottom
R5  30.28,32.62 0 top
R6  15.98,27.58 0 bottom
R7  41.7,18.68 0 bottom
R8  39.72,25.67 270 top
R9  38.32,25.68 270 top
R10  1.48,17.45 270 top
R11  26.84,21.46 180 bottom
R12  26.89,20.16 180 bottom
R13  11.72,33.82 180 top
R14  41.4,13.38 0 bottom
R15  7.01,1.53 270 top
R16  44.9,18.7 0 bottom
R17  20.39,9.16 180 bottom
R18  20.69,15.56 180 bottom
R19  44,2.28 90 bottom
R20  15.98,26.3 0 bottom
R21  45.4,2.28 270 bottom
R24  44.9,13.41 0 bottom
R25  44.9,11.91 0 bottom
R26  23.14,32.81 0 bottom
R28  22.54,31.23 0 bottom
R30  41.36,11.95 180 bottom
R31  39.89,20.21 0 top
R32  40.53,16.09 270 top
R33  42.99,33.86 0 bottom
R34  37.22,30.12 180 top
R37  1.4,25.9 270 top
R42  39.15,16.16 90 top
R44  46.65,33.86 0 bottom
R45  30.28,34.03 0 top
R46  33.48,30.12 0 top
R47  36.84,20.25 180 top
U1  5.9,3.98 270 bottom
U2  17.3,17.08 0 top
U3  15.82,7.34 0 bottom
U4  26.96,28.79 0 bottom
U10  44.8,5.38 0 bottom
U$3  [LOGO]  29.96,10.17 0 bottom
U$4  [LOGO_SIYING]  0.7,0.38 0 top
U$37  13.59,13.83 0 top
U$38  21.11,22.67 0 top
WORK  46.72,33.98 180 top

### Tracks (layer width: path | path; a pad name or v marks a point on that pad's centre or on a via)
D+
  Top 0.152: R9.1 39.03,27.15 39.06,27.15 40.3,28.39 40.9,28.39 41,28.28 | J1.A6 42.27,27.88 41.2,27.88 41,28.08 41,28.28 | J1.B6 42.27,28.88 41,28.88 41,28.28
  Top 0.172: 41.62,27.86 J1.A6
D-
  Top 0.152: J1.A7 43.12,28.36 43.2,28.28 43.2,27.58 43.2,27.46 43.1,27.36 | J1.B7 42.26,27.34 40.3,27.34 39.72,26.76 R8.1
  Top 0.172: J1.A7 42.62,28.36 | J1.B7 43.1,27.36
EAR_N
  Top 0.157: U2.41 30.82,15.08
  Top 0.172: C42.2 C23.2 35.43,17.42 35.43,18.65 35.2,18.88 34.05,18.88 33.8,18.64 33.8,17.47 C19.1 32.43,16.69 30.82,15.08
EAR_P
  Top 0.172: C5.1 C19.2 33.21,15.44 33.21,15.28 C44.2 33.03,15.3 32.95,15.38 31.99,15.38 30.69,14.08 U2.40
GND  (via drill 0.3, 0.35, 0.53)
  Top 0.152: C2.2 1.46,16.36 1.48,16.38
  Top 0.172: R45.1 29.43,34.11 27.91,34.11 C30.-
  Top 0.178: Q6.2 32.5,31.98 | 1.48,16.38 R10.2 | U2.59 18.31,29.12 18.39,29.08 U2.58
  Top 0.215: C14.1 31.32,31.27 32.03,31.98 32.5,31.98 | Q6.2 32.86,32.08 33.72,31.22 34.53,31.22 35.29,30.46 v35.29,30.21 | v22.63,13.11 23.1,12.63 23.1,8.68 | v36.46,12.95 36.46,14.45 36.99,14.98 36.99,16.16 37.49,16.67 C23.1
  Top 0.217: U2.89 6.36,5.14 6.36,6.2 | 6.36,6.2 6.36,6.3 6.5,6.44 7.71,6.44 | 6.4,6.24 6.36,6.2 | U2.91 8.25,5.14 8.25,6.3 8.11,6.44 7.71,6.44 | 7.71,6.44
  Top 0.218: C5.2 32.38,17.5 v32.13,17.5
  Top 0.254: U2.29 20.3,3.66 v20.58,3.38
  Top 0.315: C38.2 39.03,17.04 R42.2 37.96,16.92 C23.1
  Top 0.317: 9.63,32.48 C9.1 8.34,32.33 J6.P$2 | J4.P$1 5.15,5.35 5.76,5.08 U2.89 | C41.1 36.06,20.27 R47.2 36.95,19.38 v36.95,19.18 36.95,17.64 37.71,16.89 C23.1
  Top 0.318: v2.62,16.85 1.32,16.85 R10.2 | K3.2 2.74,20.78 v3,20.78
  Top 0.572: C10.1 22.27,32.33 23.3,31.3 U2.54 | C28.1 18.11,32.76 C15.1 18.18,31.79 18.41,31.56 18.41,29.58
  Bottom 0.172: U3.5 17.22,8.57 19.56,6.23 C25.2 | C32.1 19.43,14.27 18.99,14.27 v18.87,14.16
  Bottom 0.215: C13.1 7.37,5.14 U1.1 8.32,4.93 C16.2 | 13.7,30.91 v13.7,30.88
  Bottom 0.254: C29.1 19.63,11.06 18.9,11.79 v18.84,11.79
  Bottom 0.415: J1.P$3 49.54,21.68 49.54,8.79 49.32,8.57 49.32,4.41 v49.16,4.25
  Bottom 0.524: C7.2 R3.2 21.57,27.64 C18.1 23.17,27.71 C26.1 23.36,27.91 25.13,27.91 26.1,28.88 29.22,28.88 v29.62,28.47
  other vias: 4.07,33.91 3.8,32.38 4.2,30.78 5.4,30.68 11.9,31.38 10.89,32.31 12.75,32.51 9.1,30.82 4.39,27.6 9.16,27.05 17.26,2.65 0.72,8.17 1.26,7.45 0.86,3.15 3.46,1.35 4.33,0.53 9.56,22.85 25.86,19.05 25.5,33.94 31.36,20.25 32.36,21.75 35.86,23.25 33.36,23.25 30.39,29.41 30.69,28.51 34.69,23.27 31.51,25.26 46.76,29.55 47.86,25.25 15.83,3.11 25.23,7.81 32.23,14.01 35.39,29.17 23.02,24.96 15.15,24.85 28.45,33.46 31.76,12.75 9.63,3.51 31.49,29.41 38.09,31.41 2.96,9.65 24.83,11.61 4.68,2.86 13.32,11.98 2.1,31.18 7.9,30.78 3.6,29.28 15.8,33.68 15.3,34.38 22.2,26.48 19.3,25.68 19.5,24.58 25.7,33.14 29.03,7.91 29.43,5.71 27.83,3.31 25.03,3.41 22.03,3.31 48.96,31.05 48.96,27.45 42.46,9.15 31.86,0.85 33.86,5.55 26.93,7.51 9.56,15.15 44.76,6.95 47.66,5.55 44.86,8.95 40.96,0.75 38.46,0.75 11.63,1.01 41.01,26.46
  pour Top (no thermals): 0.1,34.88 -0.43,34.35 -0.43,1.91 2.1,-0.62 48.1,-0.62 50.1,1.38 50.1,34.88 49.6,35.38 0.1,35.38
  pour Bottom (no thermals): -0.4,35.88 -0.4,0.88 1.1,-0.62 50.1,-0.62 50.1,34.88 49.1,35.88
GNSS_PWR_EN  (via drill 0.3)
  Top 0.152: v1.83,21.8 1.83,21.86 0.5,23.18
  Top 0.178: R37.2 1.22,25.14 0.5,24.42 0.5,23.18
  Top 0.215: U2.20 11.3,4.33 10.83,3.85 v10.83,3.66
  Bottom 0.178: v1.83,21.8 1.5,21.48 1.5,9.72 3.07,8.15 6.43,8.15 7.15,7.43
  Bottom 0.215: 7.15,7.43 7.53,7.43 10.83,4.13 v10.83,3.66
GNSS_RXD  (via drill 0.3)
  Top 0.172: U2.50 30.4,24.08 30.99,23.5 v30.97,23.48
  Bottom 0.172: v30.97,23.48 30.97,22.88 29.55,21.46 R11.2
GNSS_TXD  (via drill 0.3)
  Top 0.172: U2.49 30.38,23.08 30.8,22.66 v30.8,21.58
  Bottom 0.172: R12.2 28.57,21.08 29.8,21.08 30.3,21.58 v30.8,21.58
GPS_ANT3V3  (via drill 0.35)
  Top 0.152: 9.92,2.29 C22.2 9.91,2.19 L1.1
  Top 0.215: v10.96,1.72 10.4,2.29 9.92,2.29
  Bottom 0.215: U1.2 8.32,3.03 C16.1 8.82,3.22 9.37,2.67 10.02,2.67 v10.96,1.72
MIC_P
  Top 0.172: 36.41,18.38 C12.2 | U2.42 30.2,16.08 31.41,17.28 31.41,17.88 31.95,18.43
  Top 0.218: 36.41,18.38 35.55,19.23 32.75,19.23 31.95,18.43
MIC_VCCOUT
  Top 0.152: 37.9,18.15 C12.1
  Top 0.218: 40.51,16.88 R32.1
  Top 0.315: C12.1 37.71,18.75 39.13,20.17 R31.1 40.55,18.79 C38.1 40.55,16.87 R32.1
N$1
  Bottom 0.172: R18.1 18.88,15.56 18.24,14.92 U3.3
N$2
  Bottom 0.152: 17.96,10.73 17.8,10.89 17.8,11.98 17.4,12.38 U3.2
  Bottom 0.172: 17.96,10.73 19.54,9.16 R17.1
N$3
  Bottom 0.152: R6.1 16.8,27.64 16.8,29.48 16.5,29.78 16.5,29.79
  Bottom 0.172: Q1.1 16.04,29.79 16.5,29.79
  Bottom 0.215: Q1.1 15.34,31.1 15.64,31.1 16.34,31.8 R4.1
N$4
  Bottom 0.152: Q2.1 40.4,15.37 41.2,16.18 41.2,18.42 R7.2
N$5
  Top 0.172: U2.52 25.3,30.48 26.53,31.7 28.59,31.7 R5.1
N$7  (via drill 0.3)
  Top 0.152: v42.9,2.78 42.24,2.12 CHR.-
  Bottom 0.152: R19.1 42.9,2.62 v42.9,2.78
N$8
  Top 0.152: 3.65,19.78 1.98,18.11 1.58,18.11 R10.1
  Top 0.172: 3.9,20.08 U2.6
  Top 0.178: 3.9,20.08 3.65,19.83 3.65,19.78
N$9
  Top 0.152: L1.2 8.35,0.77 R15.2 | 2.8,3.44 J4.P$3
  Top 0.172: R15.2 6.95,0.77 6.73,0.91 6.37,0.91 arc-45 4.57,1.66 J4.P$3 2.88,3.35
N$10  (via drill 0.3)
  Top 0.175: U2.95 28.3,27.99 26.75,26.43 26.75,22.9 v26.65,22.83
  Bottom 0.172: R12.1 26.8,20.84
  Bottom 0.218: 26.8,20.84 26.8,22.68 v26.65,22.83
N$11
  Bottom 0.152: Q5.1 44.03,15.28 42.92,14.17 41.43,14.17 R14.2
N$12  (via drill 0.3)
  Top 0.2: 26.3,26.74 26.3,23.48 v25.7,22.88
  Top 0.218: U2.96 27.3,27.59 26.3,26.74
  Bottom 0.172: v25.7,22.88 25.7,21.84 R11.1
N$13
  Top 0.152: R13.1 13.96,33.82 C8.2 14.1,33.85 arc-45 14.12,33.84 16.85,31.11 arc-45 17.3,30.02 U2.60
N$15
  Top 0.152: R13.2 10.96,34.03 9.47,34.03 C9.2 arc45 8.08,34.43 6.6,34.43 J6.P$3
N$16
  Top 0.152: U2.90 7.2,4.98 7.2,2.49 R15.1
N$17
  Top 0.152: R34.2 34.7,31.88 34.3,31.88
  Top 0.172: Q7.1 33.81,33.98 33.61,33.77 33.61,33.04 | R5.2 31.45,33.04 33.61,33.04 | 33.61,33.04 33.61,32.38
  Top 0.215: 33.61,32.38 34.11,31.88 34.3,31.88
N$18
  Top 0.172: R47.1 37.61,20.28 36.7,21.18 35.23,21.18 33.93,21.18 C41.2 32.98,20.27 32.98,20.11 30.99,18.12 30.99,17.76 30.4,17.18 29.4,17.18 U2.43
N$20
  Bottom 0.152: U10.1 44,3.93 R19.2
N$21
  Top 0.152: J10.1 39.57,4.02 41.68,6.12 41.68,13.38 41.23,13.83 41.23,14.13 41.23,18.74 41.22,18.75 41.22,19.64 R31.2
N$22
  Bottom 0.157: R28.1 23.46,31.23 24,31.77 24,32.36 | 23.9,32.46 R26.1
  Bottom 0.254: 24.19,32.19 U4.5 24.17,32.19 24,32.36 23.9,32.46
N$23
  Top 0.152: 40.1,7.02 39.9,6.82 J10.2
  Top 0.315: R42.1 39.15,15.2 41.25,13.1 41.25,8.08 40.18,7.02 40.1,7.02
N$24
  Bottom 0.172: R1.2 19.23,12.5 18.38,13.35 16.92,13.35 U3.7
N$25  (via drill 0.35)
  Top 0.152: 15.9,9.24 14.53,7.86 14.53,6.7 15.2,6.02 15.2,5.68
  Top 0.175: U2.24 15.2,5.14 15.2,5.68 | v16.4,22.58 15.9,22.08 15.9,9.24
  Bottom 0.152: v16.4,22.58 15.96,23.03 15.96,25.4 15.22,26.15 R20.2
N$26
  Top 0.172: J10.3 38.17,9.72 37.81,10.08 37.81,15.27 C42.1
N$27
  Top 0.172: J10.4 33.27,10.02 34.95,11.7 34.95,14.86 C44.1
N$29
  Top 0.152: R2.1 1.4,29.55 0.73,28.88 0.73,27.33 R37.1 1.47,26.73 7.7,26.73 8.19,27.22
  Top 0.218: U2.98 8.19,29.08 8.19,27.22
N$31
  Bottom 0.152: U10.5 45.4,3.73 R21.1
N$32
  Top 0.152: 3.07,24.31 2.53,23.77 2,23.77 | 0.5,19.68 0.5,20.48 0.74,20.72 1.7,20.72 2.48,21.49 2.48,23.77 | 0.5,14.68 1.44,13.74 C2.1
  Top 0.172: 2.48,23.77 2,23.77 K3.1 | 4.64,25.18 U2.1
  Top 0.175: 3.07,24.31 3.93,25.18 4.64,25.18
  Top 0.178: 0.5,19.68 0.5,14.68
N$35
  Top 0.152: Q7.3 38.51,32.98 39.21,32.98 40.1,33.87 NET.-
N$36  (via drill 0.3)
  Top 0.152: v44.8,33.88 44.7,33.98 41.72,33.98 NET.+
  Bottom 0.152: v44.8,33.88 44.78,33.86 R33.1
N$37
  Top 0.152: R46.2 33.37,30.99 32.13,30.99 31.74,30.6 30.54,30.6 30.26,30.88 30.26,32.53 | R45.2 30.8,33.8 30.79,33.8
  Top 0.172: Q6.1 32.44,34.03 R45.2
  Top 0.178: 31.03,34.03 30.79,33.8 30.26,33.26 30.26,32.53
N$39
  Top 0.152: 36.5,33.02 36.94,33.02 37.69,32.28 39.8,32.28 40.78,33.26 44.4,33.26 45.35,33.26 45.98,33.89 45.98,33.96 WORK.-
  Top 0.172: 36.5,33.02 Q6.3
N$40  (via drill 0.3)
  Top 0.152: v48.4,33.78 48.33,33.83 47.68,33.78 WORK.+
  Bottom 0.152: R44.1 48.32,33.86 v48.4,33.78
N$41  (via drill 0.35)
  Top 0.152: R46.1 32.68,30.08 29.3,30.08 28.9,29.68 28.9,29.58 28.9,27.98 27.1,26.18 27.1,23.38 27.25,23.23 27.25,22.53 26.95,22.23 23.75,22.23 22.9,23.08 v22.9,23.58 | 11.3,26.6 11.9,26 18.4,26 18.45,25.96 18.6,25.8 18.6,23.98 v19,23.58
  Top 0.178: U2.66 11.3,26.6
  Bottom 0.152: v22.9,23.58 22.3,24.18 20.2,24.18 19.6,23.58 v19,23.58
RX_H  (via drill 0.35)
  Top 0.152: 44.6,17.5 44.7,17.4 | J9.2 42.81,17.4 v42.7,17.5
  Top 0.175: J9.2 44.7,17.4 45.33,17.4
  Bottom 0.152: v42.7,17.5 42.78,17.5 | Q2.3 42.38,17.18 v42.7,17.5 | v42.7,17.5 43.2,17 43.2,16.6 43.62,16.18 44.8,16.18 45.3,15.68 45.3,13.77 R24.1
RXD  (via drill 0.3)
  Top 0.152: 3.34,12.45 1.6,12.45 1.1,11.95 1.1,9.28 2.35,8.04 4.8,8.04 4.98,8.04 5.43,7.58 v11.2,7.58
  Top 0.178: U2.10 4.28,16.08 3.85,15.66 3.85,12.96 3.34,12.45
  Bottom 0.152: v11.2,7.58 11.3,7.48 11.3,6.78 16.4,1.68 28.11,1.68 29.21,2.78 33.8,2.78 33.9,2.78 34.4,2.29 37.61,2.29 38.2,2.88 39.44,4.11 39.44,10.61 39.44,10.79 R30.1 39.5,13.05 39.5,16.3 Q2.2
SIM1_CLK  (via drill 0.3)
  Top 0.172: 23.6,7.28 23.6,14.81 22.76,15.66 v22.66,15.66
  Top 0.215: 23.6,7.28 23.6,6.8 23.3,6.5 U2.32
  Bottom 0.152: v22.66,15.66 22.56,15.56 R18.2
  Bottom 0.172: R18.2 C27.2
SIM1_DATA  (via drill 0.3)
  Top 0.152: U2.31 22.3,5.73 22.5,5.89 | 22.5,8.48 23,7.98 23,7.08 22.5,6.58
  Top 0.172: v22.34,11.88 22.5,11.71 22.5,8.48 | 22.5,6.58 22.5,5.89
  Bottom 0.172: C32.2 R1.1 21.72,12.5 v22.34,11.88
SIM1_RST  (via drill 0.3)
  Top 0.172: v24.4,7.08 24.3,6.98 U2.33
  Bottom 0.172: v24.4,7.08 24.13,7.08 22.05,9.16 R17.2 C29.2
TX_H  (via drill 0.35)
  Top 0.152: 44.73,19.25 43.88,19.25 43.6,18.98 44.5,18.98 44.7,19.18 44.7,19.48 46.1,19.48 46.4,19.18 v46.4,17.38
  Top 0.178: J9.1 44.73,19.25
  Bottom 0.152: R25.1 46.38,12.62 46.38,15.97 Q5.3 46.18,17.16 v46.4,17.38
TXD  (via drill 0.3)
  Top 0.152: 3.42,13.28 2.91,12.77 1.4,12.77 0.79,12.16 0.79,9.1 2.24,7.65 4.5,7.65 4.94,7.65 5.4,7.18 9.6,7.18
  Top 0.172: v10.4,6.98 10.3,7.08 9.7,7.08 9.6,7.18
  Top 0.178: U2.9 4.58,17.08 3.42,15.92 3.42,13.28
  Bottom 0.152: Q5.2 45.47,18.38 46.08,18.38 45.96,18.5 | 45.45,18.7 R16.1 45.67,18.79 45.96,18.5 | 45.96,18.5 46.26,18.5 47.31,17.45 47.31,15.4 46.9,14.99 46.9,11.08 46.1,10.27 43.91,10.27 43.9,10.28 41.1,10.28 40.34,9.52 40.34,3.52 38.4,1.58 31.14,1.58 30.8,1.25 16.14,1.25 v10.4,6.98
USB_D+  (via drill 0.35)
  Top 0.152: R9.2 38.52,24.72 38.52,23.9 v38.5,23.88 | v34.3,13.18 34.5,12.98 34.5,12.08 33.57,11.15 31.47,11.15 31.1,10.78 31.1,6.68 30.6,6.18 30.6,3.69 29.1,2.19 18.7,2.19 18.3,2.59 U2.27
  Bottom 0.152: v34.3,13.18 38.5,17.38 38.5,18.88
  Bottom 0.175: v38.5,23.88 38.5,18.88
USB_D-  (via drill 0.35)
  Top 0.152: R8.2 39.9,24.73 v39.9,23.88 | v33.7,12.48 32.8,11.58 31.37,11.58 30.67,10.88 30.67,9.08 30.67,6.84 30.2,6.37 30.2,3.89 28.89,2.58 19.3,2.58 U2.28
  Top 0.175: 19.3,3.95 U2.28
  Bottom 0.152: v33.7,12.48 34.53,12.48 39,16.96
  Bottom 0.175: v39.9,23.88 39,22.98 39,16.96
USIM1_VDD  (via drill 0.3)
  Top 0.315: v22.28,7.51 21.68,6.91 21.68,5.99 21.3,5.62 U2.30
  Bottom 0.315: C20.1 22.04,7.75 v22.28,7.51
  Bottom 0.317: U3.1 17.52,9.84 19.39,7.96 19.42,7.96 | 19.42,7.96 C25.1 | C20.1 19.92,7.75 19.71,7.96 19.51,7.96 19.42,7.96
VBAT_IN  (via drill 0.3)
  Top 0.157: 19.64,32.56 19.64,32.62 C15.2 19.64,32.76 C28.2 21.11,33.99 v21.3,34.18 | v20.5,33.68 20.6,33.58 v20.6,32.58 | v21.3,34.18 v21.3,33.08 | v21.3,34.18 21.37,34.11 C10.2 23.77,34.11 24.11,33.77 C30.+ | U2.55 21.69,29.08 21.69,29.75 21.61,29.68 21.39,29.68 21.38,29.55 U2.56 | 20.7,29.08 U2.57
  Top 0.517: U2.56 20.7,29.08 | U2.56 21.05,29.08 20.58,29.55 | U2.56 21.07,29.32 20.44,29.32 | 20.49,29.37 20.49,29.27 U2.57 U2.56 | U2.56 U2.55
  Top 0.524: U2.57 20.44,29.32 20.58,29.55 20.8,29.95 20.8,31.39 19.64,32.56
  Bottom 0.152: v21.3,34.18 21.68,34.56 30.53,34.56 30.9,34.18 39.6,34.18 39.8,33.98 42.11,33.98 R33.2 42.93,34.56 45.19,34.56 R44.2
  Bottom 0.157: v20.5,33.68 21,34.18 v21.3,34.18 | v21.3,33.08 20.6,32.38 20.4,32.38
  Bottom 0.172: v21.3,33.08 v21.3,34.18
  Bottom 0.532: 20.4,31.46 20.09,31.15 B1.1 20.1,33.28 v20.5,33.68
  Bottom 0.832: 20.55,32.53 20.5,32.48 | v20.6,32.58 20.55,32.53 | 20.19,32.17 20.4,32.38 20.5,32.48 | 20.09,31.21 B1.1 | v21.3,33.08 20.75,32.53 20.55,32.53 | v21.3,34.18 20.8,33.68 v20.5,33.68 20.5,32.48
VBAT_VCC1  (via drill 0.35)
  Top 0.152: v35.71,8.08 v35.7,8.07 v35.7,7.18 v35.7,6.18 | 44,3.98 44.1,3.88 J3.1 46.2,3.88
  Top 1.015: 41.65,3.08 40.75,2.18
  Top 1.152: 40.75,2.28 40.75,2.18 | 41.65,3.08 v41.65,3.58 | v41.65,3.58 41.65,3.98 | v41.7,4.58 41.7,3.64 v41.65,3.58
  Top 1.252: 44,3.98 41.65,3.98
  Top 1.515: 40.75,2.28 38.6,2.28 37.4,2.28 37.4,4.89 35.7,6.59 v35.7,7.18
  Bottom 0.815: U10.3 43.5,7.38 C21.1 42.61,7.58 42.6,7.58
  Bottom 1: Q1.3 13.49,28.76
  Bottom 1.152: 42.6,7.58 42.2,7.58 41.7,7.08 v41.7,4.58
  Bottom 1.515: 13.49,28.76 11.45,26.72 11.45,20.34 12.5,19.28 23.1,19.28 35.7,6.68 v35.7,6.18
VBUS  (via drill 0.3, 0.35)  (1 unrouted)
  Top 0.152: CHR.+ 44.77,2.78 48.2,2.78 48.5,3.08 48.5,6.88 v48.35,6.88 | J1.B9 J1.A4 42.4,25.68 42.7,25.68 | J1.A9 42.28,30.46 J1.B4 | J1.A9 42.41,30.54 | J1.A9 42.08,30.46 41.1,30.46 | v31.8,27.98 31.9,28.08 v32.6,28.08 32.77,27.91 32.77,27.16 31.88,27.16 v31.8,27.08
  Top 0.178: v31.8,27.08 v31.8,27.98
  Top 0.515: 37,24.08 38,23.08 40.4,23.08 40.8,23.48 40.8,25.08 41.35,25.62 42.65,25.62 42.7,25.68
  Top 0.524: 42.07,25.68 42.7,25.68 43.1,25.68 44,26.58 44,26.68 | v44.4,29.78 43.9,29.78 43.15,30.54 42.41,30.54 | 42.28,30.46 41.1,30.46 40.78,30.46 40.4,30.09
  Top 0.532: C4.+ 33.14,27.72 v32.68,27.25 32.5,27.08 v31.8,27.08 | v31.8,27.98 32.5,27.98 v32.6,28.08 35.62,28.08 35.8,27.89 35.9,27.79 | C1.2 32.69,26.05 32.69,26.36 32.77,26.36 C1.2
  Top 0.572: v44.3,26.68 44.4,26.78 | v44.3,26.68 44,26.68 | v44.3,26.68 v45.2,26.68 | v45.3,29.68 45.2,29.78 v44.4,29.78
  Top 0.832: v32.68,27.25 32.77,27.16 C1.2
  Top 1: 36.94,27.28 36.94,24.14 37,24.08
  Top 1.517: C4.+ 35.02,27.79 35.9,27.79 | 35.8,27.89 38.2,27.89 38.2,27.99
  Top 1.524: 38.2,27.89 40.4,30.09 40.4,30.18
  Bottom 0.152: R20.1 15.49,27.55 15.49,27.56 15.39,27.57 | 15.39,27.57 13.99,27.57 12.6,26.18 12.6,20.88 13.02,20.47 21.9,20.47 24.36,22.92 24.36,24.84 24.75,25.23 25.55,25.23 | 15.39,27.57 R6.2 | 26.83,25.39 U4.1 26.8,25.23 25.55,25.23 | 25.8,25.38 25.7,25.38 25.55,25.23 | v48.35,6.88 47.79,6.33 U10.4
  Bottom 0.178: U4.2 27.9,27.09
  Bottom 0.572: v45.2,26.68 45.2,29.58 v45.3,29.68 | v32.6,28.08 32.68,28.01 v32.68,27.25 | v31.8,27.98 v31.8,27.08 | 27.9,27.09 29.5,27.09 | 29.92,27.29 29.5,27.29 29.5,27.09 | 29.5,27.09 29.5,25.58 29.3,25.38 26.97,25.38 U4.1
  Bottom 0.615: C6.2 46.98,7.56 | 46.98,7.56 46.3,6.88 46.1,6.88 | 46.98,7.56 46.8,7.74 46.8,8.18 46.47,8.18 | 46.47,8.18 | 46.47,8.18 45.9,8.18 45.9,7.66 46.1,7.46
  Bottom 1.152: v45.2,26.68 45.2,23.38 48.4,20.18 48.4,8.98 46.98,7.56 | 46.1,7.46 46.1,6.88 U10.4
  Bottom 1.516: 32.2,27.08 26.97,27.08 U4.2
VCC  (via drill 0.35)
  Top 0.215: v43.4,11.08 43.05,11.44 43.05,14.89 43.56,15.4 J9.3
  Bottom 0.215: R24.2 43.82,13.09 | R25.2 43.4,11.17 v43.4,11.08
  Bottom 0.318: 43.82,13.09 43.82,11.49 v43.4,11.08
VCC_4V  (via drill 0.35)
  Top 0.215: v11.8,17.48 11.8,7.85 11.82,7.83 11.82,7.33 10.86,6.37 9.93,6.37 9.45,6.84 4.89,6.84 v4.79,6.74
  Bottom 0.157: C18.2 21.64,31.1 R28.2
  Bottom 0.178: 21.5,29.36 21.3,29.16 R3.1 | C18.2 23.17,29.49 C26.2 23.09,29.16 C7.1
  Bottom 0.215: v11.8,17.48 11.78,17.5 11.78,18.56 10.3,20.04 10.3,28.88 14.46,33.03 17.65,33.03 18.32,32.37 B1.2 18.57,30.87 18.57,30.8 | v4.79,6.74 5.35,6.18 C13.2 5.84,5.17 U1.3
  Bottom 1.152: Q1.2 18.57,30.8
  Bottom 1.157: 23.73,29.36 C26.2 21.5,29.36 | 21.3,29.16 C7.1 | 18.47,30.97 B1.2
  Bottom 1.557: U4.4 24.86,30.49 23.73,29.36
  Bottom 1.572: C7.1 18.57,30.8
VDD_1V8  (via drill 0.3, 0.35)
  Top 0.152: v29.8,1.98 29.8,1.96 29.5,1.66 | v41.8,20.18 41.9,20.08 41.63,19.81 41.63,14.05 42.1,13.58 42.1,11.19 v42.3,10.98
  Top 0.172: v2.45,28.18 2.38,28.11 R2.2
  Top 0.215: 11.24,19.05 9.2,19.05 8.39,18.24 8.39,11.52 v8.63,11.28
  Top 0.218: 29.5,1.66 13.43,1.66 v13,2.08
  Top 0.315: U2.97 26.3,30.58 26.9,31.18 29.4,31.18 C14.2 | v24.3,26.78 24.49,26.78 24.6,26.89 | v3.06,11.42 3,11.36 C3.2
  Top 0.317: U2.97 26.31,27.69 25.5,26.89 24.6,26.89 24.52,26.81
  Top 0.318: U2.15 3.4,11.08 v3.06,11.42
  Top 0.322: 11.24,19.05 v13.34,21.15
  Bottom 0.152: R16.2 44.12,18.68 R7.1 41.8,19.34 v41.8,20.18 | R14.1 42.12,13.34 R30.2 | v29.8,1.98 38,1.98 39.9,3.88 39.9,9.73 R30.2 | R30.2 42.3,11.77 v42.3,10.98
  Bottom 0.178: v2.45,28.18 2.55,28.18 3.65,27.08 3.65,11.98
  Bottom 0.215: 3.6,11.28 3.85,11.28 3.7,11.42 v3.06,11.42 3.96,11.42 4.1,11.28 | 3.6,11.28 3.2,11.28 | 3.65,11.98 3.65,11.32 3.6,11.28 | v8.63,11.28 8.5,11.41
  Bottom 0.218: v13,2.08 13,3.48 8.7,7.78
  Bottom 0.315: v24.3,26.78 23.9,26.38 23.9,23.18 21.67,20.95
  Bottom 0.318: 21.67,20.95 13.54,20.95 v13.34,21.15 | 8.7,11.28 8.7,7.78 | 8.7,11.28 4.1,11.28 3.85,11.28 | v3.06,11.42 3.2,11.28 | v8.63,11.28 8.7,11.35 8.7,11.28
VDD_AUX3V  (via drill 0.3, 0.35)
  Top 0.215: v35.9,11.88 35.8,11.88 34.28,10.35 34.28,7.01 33.93,6.66 31.78,6.66 31.1,5.98 31.1,1.96 30.22,1.08 12.9,1.08 12,1.98 v12,2.18 | 6.6,21.38 6.6,8.98 7.34,8.24 v7.34,8.22 | v38.47,13.98 38.41,14.04 38.41,15.89 38.7,16.18 39.7,16.18 40.53,15.35 R32.2
  Top 0.218: v7.2,21.98 6.6,21.38
  Top 0.317: U2.99 v7.3,27.48
  Bottom 0.152: C11.2 7.3,25.71 7.3,25.88
  Bottom 0.215: v35.9,11.88 35.97,11.81 36.52,11.81 38.47,13.76 v38.47,13.98
  Bottom 0.218: C11.2 7.4,25.61 7.4,22.18 v7.2,21.98 | v7.34,8.22 7.47,8.22 12,3.68 v12,2.18
  Bottom 0.317: 7.3,25.88 v7.3,27.48
(copper drawn outside any net)
  shapes: Bottom area x8, Top area x9

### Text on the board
tPlace: TX | RX | VCC | GND
bPlace: Crowtail-4G SIM-A7670C V1.0 / www.elecrow.com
